(* Logix 5000 AddOnInstructionDefinition export Banner_S15C_MGN_PD_v4; software revision 33.00 *)

TYPE Banner_S15C_MGN_PDIO_v4 :   // UDT with all of the variables needed to control an IO-Link S15C MGN.
STRUCT
   Read : Banner_S15C_MGN_Read_DS_v4;   // English Data Set
   Write : Banner_S15C_MGN_Write_DS_v4;   // Metric Data Set
   DTI : SINT[32];   // Array with Raw Process data being transferred into AOI.
   DTO : SINT[32];   // Array with Raw Process data being transferred into AOI.
END_STRUCT
END_TYPE

TYPE Banner_S15C_MGN_Read_DS_v4 :
STRUCT
   Read_Data_Set : SINT;
   Read_Success : SINT;
   Write_Success : SINT;
   Register_Verify : SINT;
   Counter_Value : INT;
   Read_Regs : DINT[16];
END_STRUCT
END_TYPE

TYPE Banner_S15C_MGN_Write_DS_v4 :
STRUCT
   Set_to_Read : SINT;
   Write_Regs : DINT[16];
END_STRUCT
END_TYPE

ADD_ON_INSTRUCTION Banner_S15C_MGN_PD_v4   (* revision 4.0, vendor Banner Engineering *)
// AOI that used with the S15C MGN sensor.
VAR_IN_OUT
   PD : Banner_S15C_MGN_PDIO_v4; {required}
END_VAR
VAR_INPUT
   Byte_Swap : BOOL; {required}
END_VAR
VAR
   TempR : SINT[32]; {access None}
   W_Index : SINT; {access None}
   DTI_Index : SINT; {access None}
   R_Index : SINT; {access None}
   DTO_Index : SINT; {access None}
   R_Data_Update : BOOL; {access None}
   TempW : SINT[32]; {access None}
   W_Data_Update : BOOL; {access None}
END_VAR

ROUTINE Logic   (* ladder *)
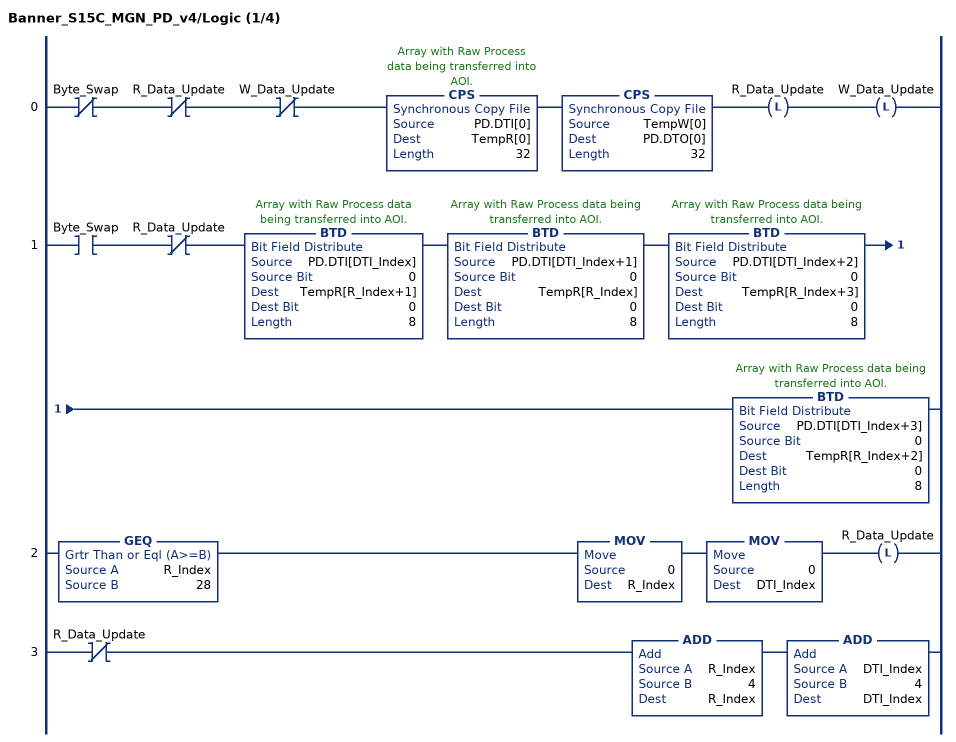
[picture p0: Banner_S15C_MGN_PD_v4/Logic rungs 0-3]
   0: XIO(Byte_Swap)XIO(R_Data_Update)XIO(W_Data_Update)CPS(PD.DTI[0],TempR[0],32)CPS(TempW[0],PD.DTO[0],32)OTL(R_Data_Update)OTL(W_Data_Update);
   1: XIC(Byte_Swap)XIO(R_Data_Update)BTD(PD.DTI[DTI_Index],0,TempR[R_Index+1],0,8)BTD(PD.DTI[DTI_Index+1],0,TempR[R_Index],0,8)BTD(PD.DTI[DTI_Index+2],0,TempR[R_Index+3],0,8)BTD(PD.DTI[DTI_Index+3],0,TempR[R_Index+2],0,8);
   2: GEQ(R_Index,28)MOV(0,R_Index)MOV(0,DTI_Index)OTL(R_Data_Update);
   3: XIO(R_Data_Update)ADD(R_Index,4,R_Index)ADD(DTI_Index,4,DTI_Index);
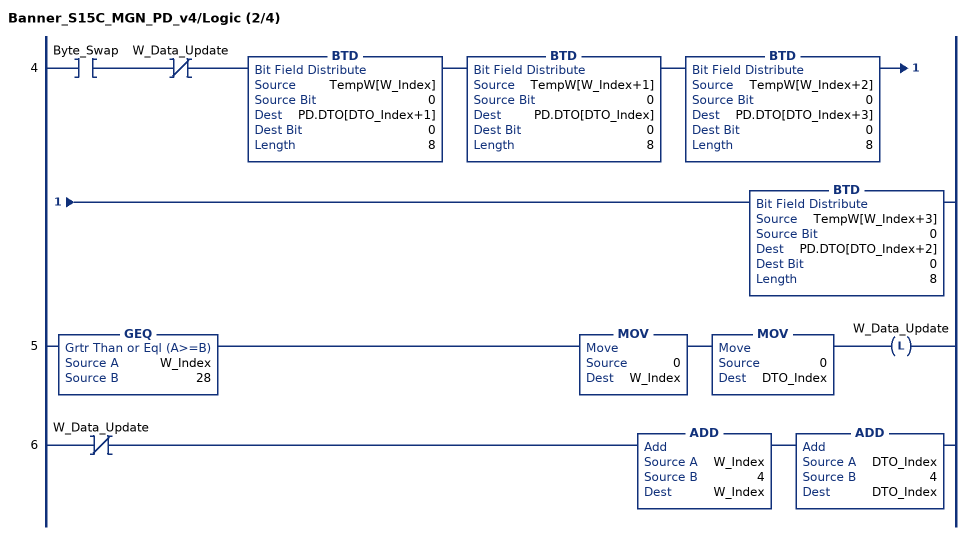
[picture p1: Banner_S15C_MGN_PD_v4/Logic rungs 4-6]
   4: XIC(Byte_Swap)XIO(W_Data_Update)BTD(TempW[W_Index],0,PD.DTO[DTO_Index+1],0,8)BTD(TempW[W_Index+1],0,PD.DTO[DTO_Index],0,8)BTD(TempW[W_Index+2],0,PD.DTO[DTO_Index+3],0,8)BTD(TempW[W_Index+3],0,PD.DTO[DTO_Index+2],0,8);
   5: GEQ(W_Index,28)MOV(0,W_Index)MOV(0,DTO_Index)OTL(W_Data_Update);
   6: XIO(W_Data_Update)ADD(W_Index,4,W_Index)ADD(DTO_Index,4,DTO_Index);
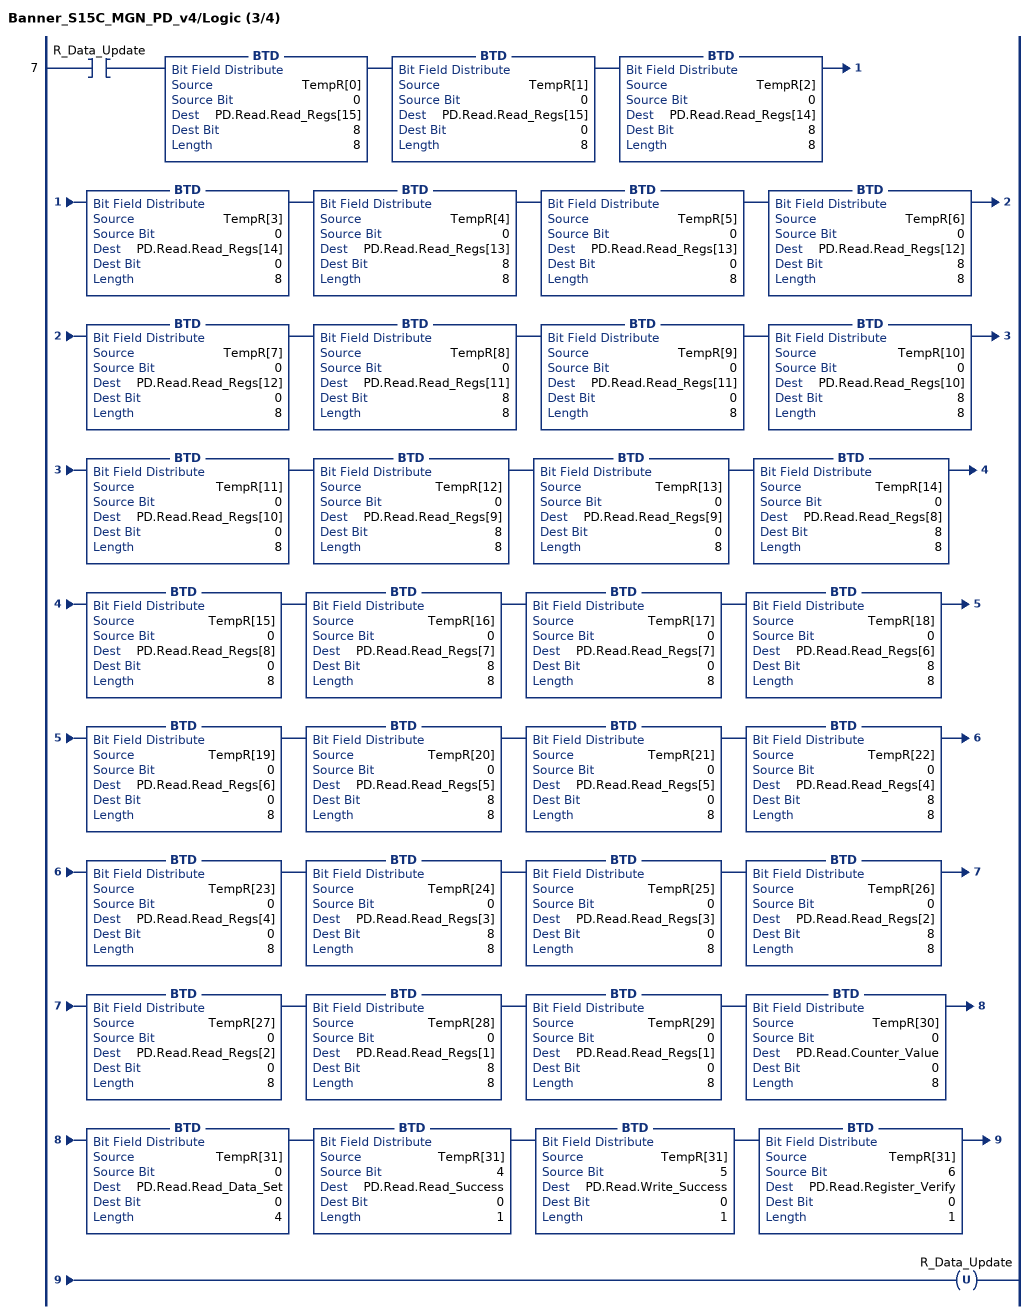
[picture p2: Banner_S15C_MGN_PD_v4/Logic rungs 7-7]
   7: XIC(R_Data_Update)BTD(TempR[0],0,PD.Read.Read_Regs[15],8,8)BTD(TempR[1],0,PD.Read.Read_Regs[15],0,8)BTD(TempR[2],0,PD.Read.Read_Regs[14],8,8)BTD(TempR[3],0,PD.Read.Read_Regs[14],0,8)BTD(TempR[4],0,PD.Read.Read_Regs[13],8,8)BTD(TempR[5],0,PD.Read.Read_Regs[13],0,8)BTD(TempR[6],0,PD.Read.Read_Regs[12],8,8)BTD(TempR[7],0,PD.Read.Read_Regs[12],0,8)BTD(TempR[8],0,PD.Read.Read_Regs[11],8,8)BTD(TempR[9],0,PD.Read.Read_Regs[11],0,8)BTD(TempR[10],0,PD.Read.Read_Regs[10],8,8)BTD(TempR[11],0,PD.Read.Read_Regs[10],0,8)BTD(TempR[12],0,PD.Read.Read_Regs[9],8,8)BTD(TempR[13],0,PD.Read.Read_Regs[9],0,8)BTD(TempR[14],0,PD.Read.Read_Regs[8],8,8)BTD(TempR[15],0,PD.Read.Read_Regs[8],0,8)BTD(TempR[16],0,PD.Read.Read_Regs[7],8,8)BTD(TempR[17],0,PD.Read.Read_Regs[7],0,8)BTD(TempR[18],0,PD.Read.Read_Regs[6],8,8)BTD(TempR[19],0,PD.Read.Read_Regs[6],0,8)BTD(TempR[20],0,PD.Read.Read_Regs[5],8,8)BTD(TempR[21],0,PD.Read.Read_Regs[5],0,8)BTD(TempR[22],0,PD.Read.Read_Regs[4],8,8)BTD(TempR[23],0,PD.Read.Read_Regs[4],0,8)BTD(TempR[24],0,PD.Read.Read_Regs[3],8,8)BTD(TempR[25],0,PD.Read.Read_Regs[3],0,8)BTD(TempR[26],0,PD.Read.Read_Regs[2],8,8)BTD(TempR[27],0,PD.Read.Read_Regs[2],0,8)BTD(TempR[28],0,PD.Read.Read_Regs[1],8,8)BTD(TempR[29],0,PD.Read.Read_Regs[1],0,8)BTD(TempR[30],0,PD.Read.Counter_Value,0,8)BTD(TempR[31],0,PD.Read.Read_Data_Set,0,4)BTD(TempR[31],4,PD.Read.Read_Success,0,1)BTD(TempR[31],5,PD.Read.Write_Success,0,1)BTD(TempR[31],6,PD.Read.Register_Verify,0,1)OTU(R_Data_Update);
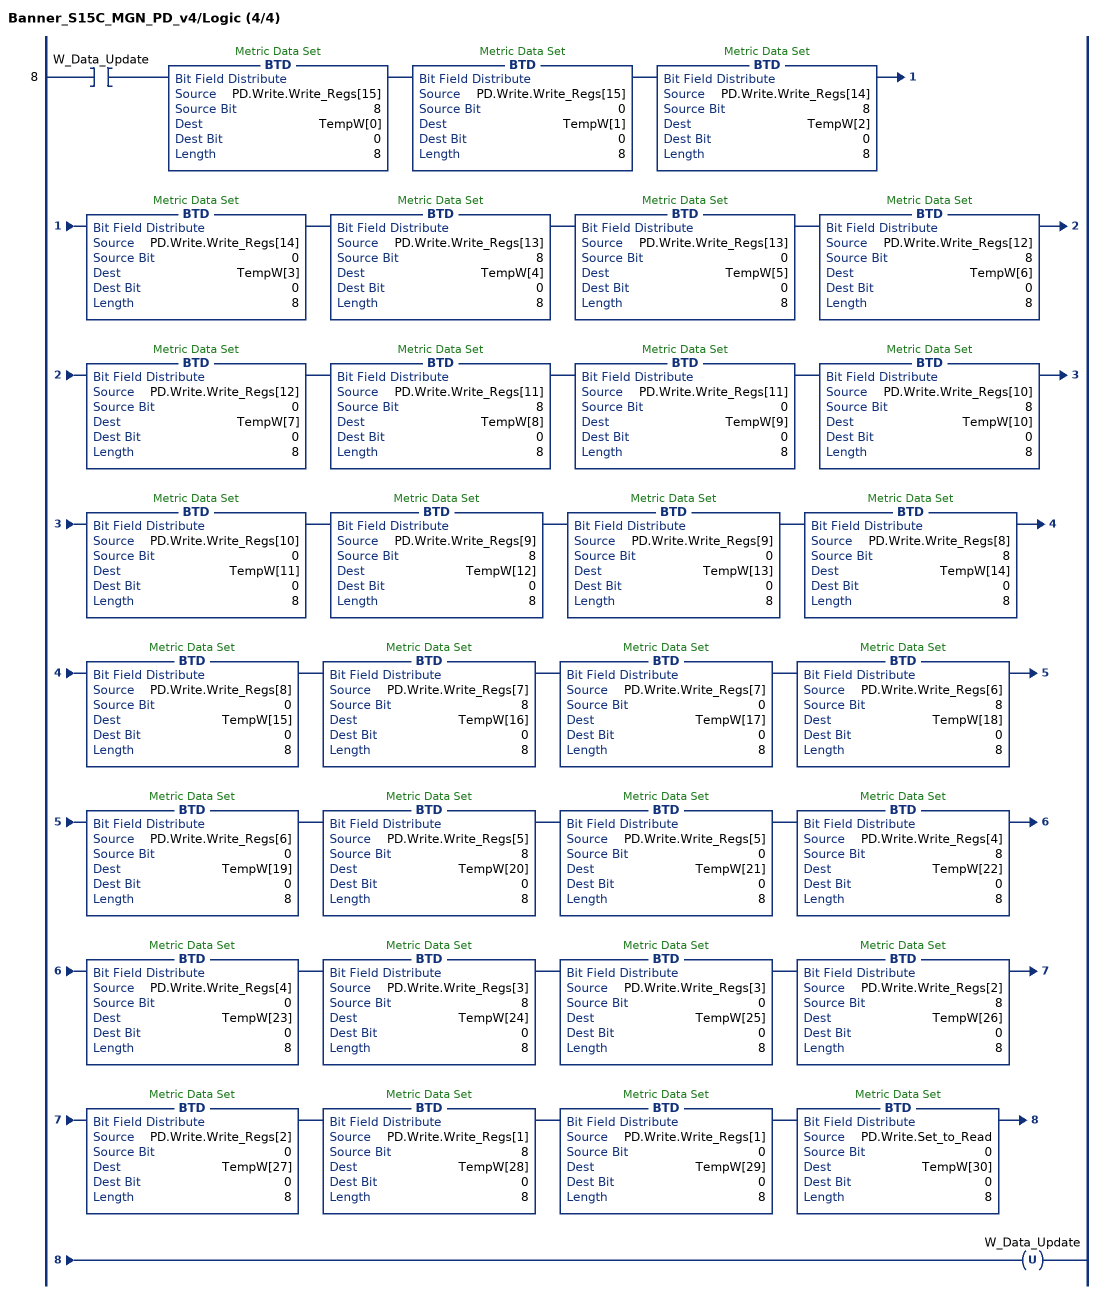
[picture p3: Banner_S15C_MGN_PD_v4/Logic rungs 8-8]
   8: XIC(W_Data_Update)BTD(PD.Write.Write_Regs[15],8,TempW[0],0,8)BTD(PD.Write.Write_Regs[15],0,TempW[1],0,8)BTD(PD.Write.Write_Regs[14],8,TempW[2],0,8)BTD(PD.Write.Write_Regs[14],0,TempW[3],0,8)BTD(PD.Write.Write_Regs[13],8,TempW[4],0,8)BTD(PD.Write.Write_Regs[13],0,TempW[5],0,8)BTD(PD.Write.Write_Regs[12],8,TempW[6],0,8)BTD(PD.Write.Write_Regs[12],0,TempW[7],0,8)BTD(PD.Write.Write_Regs[11],8,TempW[8],0,8)BTD(PD.Write.Write_Regs[11],0,TempW[9],0,8)BTD(PD.Write.Write_Regs[10],8,TempW[10],0,8)BTD(PD.Write.Write_Regs[10],0,TempW[11],0,8)BTD(PD.Write.Write_Regs[9],8,TempW[12],0,8)BTD(PD.Write.Write_Regs[9],0,TempW[13],0,8)BTD(PD.Write.Write_Regs[8],8,TempW[14],0,8)BTD(PD.Write.Write_Regs[8],0,TempW[15],0,8)BTD(PD.Write.Write_Regs[7],8,TempW[16],0,8)BTD(PD.Write.Write_Regs[7],0,TempW[17],0,8)BTD(PD.Write.Write_Regs[6],8,TempW[18],0,8)BTD(PD.Write.Write_Regs[6],0,TempW[19],0,8)BTD(PD.Write.Write_Regs[5],8,TempW[20],0,8)BTD(PD.Write.Write_Regs[5],0,TempW[21],0,8)BTD(PD.Write.Write_Regs[4],8,TempW[22],0,8)BTD(PD.Write.Write_Regs[4],0,TempW[23],0,8)BTD(PD.Write.Write_Regs[3],8,TempW[24],0,8)BTD(PD.Write.Write_Regs[3],0,TempW[25],0,8)BTD(PD.Write.Write_Regs[2],8,TempW[26],0,8)BTD(PD.Write.Write_Regs[2],0,TempW[27],0,8)BTD(PD.Write.Write_Regs[1],8,TempW[28],0,8)BTD(PD.Write.Write_Regs[1],0,TempW[29],0,8)BTD(PD.Write.Set_to_Read,0,TempW[30],0,8)OTU(W_Data_Update);
END_ROUTINE
END_ADD_ON_INSTRUCTION
